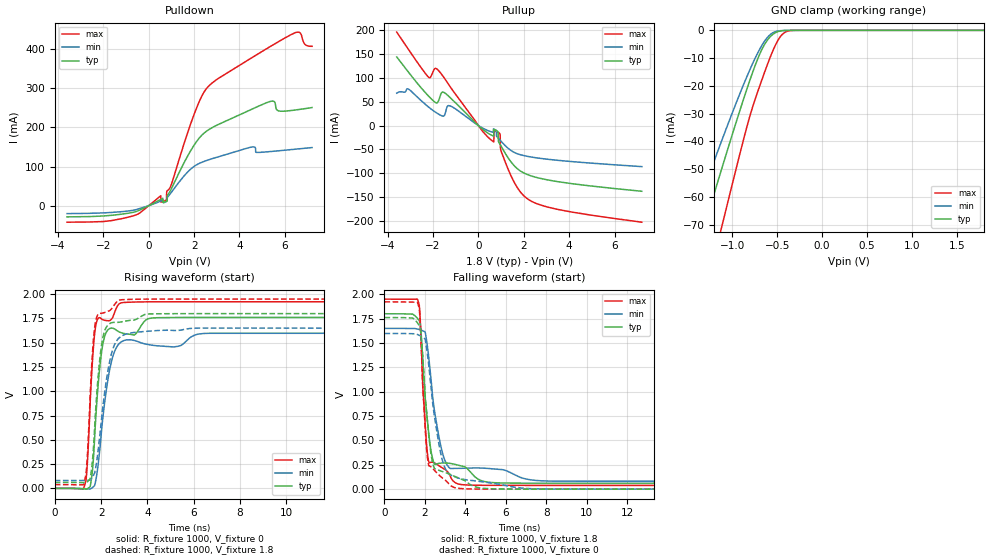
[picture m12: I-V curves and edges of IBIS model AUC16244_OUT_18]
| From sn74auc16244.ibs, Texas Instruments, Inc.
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[Model]   AUC16244_OUT_18
Model_type  3-state
Enable   Active-Low
Vref =   0
Rref =   1000
Cref =   30p
Vmeas =   0.9
| variable   typ   min   max
C_comp   5.46pF   4.88pF   5.67pF
| C_pullup   6.28pF   1.00pF   11.78pF
| C_pulldown   6.14pF   1.75pF   14.74pF
| C_tri-state   5.46pF   4.88pF   5.67pF
[Temperature Range]   40   100   -40
| Ambient temperature   25   85   -40
[Voltage range]   1.8   1.65   1.95
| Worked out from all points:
|   slope of the pulldown table from 0 to 0.27 V, typ, clamps not added: 34.2 ohm
|   slope of the pullup table from 0 to 0.27 V, typ, clamps not added: 24.9 ohm
|   GND clamp passes 1 mA (typ) near -0.53 V on its own axis
|   rising waveform, R_fixture 1000, V_fixture 0: 20-80 % time 343ps typ, 511ps min, 262ps max; typ from 0 V to 1.76 V
|   falling waveform, R_fixture 1000, V_fixture 1.8: 20-80 % time 430ps typ, 642ps min, 291ps max; typ from 1.8 V to 0.061 V
|   rising waveform, R_fixture 1000, V_fixture 1.8: 20-80 % time 339ps typ, 522ps min, 256ps max; typ from 0.061 V to 1.8 V
|   falling waveform, R_fixture 1000, V_fixture 0: 20-80 % time 432ps typ, 649ps min, 291ps max; typ from 1.76 V to 0 V
[GND Clamp]
| AUC16244_OUT_18
|   Voltage   I(typ)   I(min)   I(max)
-3.6V     -322.9mA   -271.3mA   -392.8mA
-1.48V    -89.14mA   -71.99mA   -118.6mA
-1.435V   -84.24mA   -67.93mA   -112.7mA
-1.3V     -69.59mA   -55.85mA   -94.97mA
-1.15V    -53.49mA   -42.68mA   -75.27mA
-1.1V     -48.18mA   -38.36mA   -68.71mA
-830mV    -20.57mA   -16.22mA   -34.06mA
-690mV    -8.335mA   -6.605mA   -19.75mA
-565mV    -1.951mA   -1.255mA   -8.764mA
-490mV    -463.9uA   -245.9uA   -3.576mA
-425mV    -91.38uA   -54.15uA   -985.3uA
1.8V      674.7pA    45.17nA    747.9pA
[Pulldown]
| AUC16244_OUT_18
|   Voltage   I(typ)   I(min)   I(max)
-3.6V     -28.49mA   -20.22mA   -42.08mA
-1.155V   -21.32mA   -15.05mA   -32.66mA
530mV     16.28mA    11.83mA    25.26mA
780mV     11.06mA    10.81mA    14.1mA
800mV     11.7mA     11.72mA    36.72mA
1.955V    150.3mA    98.42mA    225.9mA
2.625V    193.2mA    116.8mA    304mA
4.56V     246.5mA    149.9mA    378.1mA
5.38V     266.4mA    138.3mA    406.9mA
5.71V     242.1mA    140mA      418.2mA
6.445V    244.1mA    144.1mA    441.1mA
7.2V      250.4mA    148.3mA    406.7mA
[Pullup]
| AUC16244_OUT_18
|   Voltage   I(typ)   I(min)   I(max)
-3.6V     143.4mA    67.81mA    195.5mA
-2.21V    62.22mA    39.25mA    101.7mA
-1.955V   50.53mA    30.07mA    117.2mA
-1.505V   68.89mA    20.87mA    99.46mA
-1.25V    58.62mA    41.27mA    81.57mA
405mV     -15.38mA   -10.2mA    -23.47mA
835mV     -11.64mA   -24.19mA   -13.09mA
930mV     -37.45mA   -29.05mA   -16.21mA
980mV     -41.44mA   -31.73mA   -49.64mA
1.31V     -67.6mA    -47.58mA   -91.39mA
2.115V    -101.6mA   -63.91mA   -151.5mA
7.2V      -137.4mA   -85.82mA   -202mA
[Ramp]
| AUC16244_OUT_18
| variable   typ   min   max
dV/dt_r   1.06/3.53E-10   0.96/5.21E-10   1.16/2.72E-10
dV/dt_f   1.04/4.39E-10   0.94/6.57E-10   1.15/2.96E-10
R_load = 1000
[Rising Waveform]
| AUC16244_OUT_18
R_fixture =   1000
C_fixture =   0
L_fixture =   0
V_fixture =   0
V_fixture_min = 0
V_fixture_max = 0
|   Time   V(typ)   V(min)   V(max)
0s        9.675nV    33.63nV    1.209nV
1.325ns   -7.242mV   -3.423mV   61.54mV
1.55ns    46.88mV    -3.891mV   988.5mV
1.72ns    513.6mV    28.82mV    1.59V
1.915ns   1.179V     333.7mV    1.759V
2.13ns    1.545V     838.7mV    1.733V
2.47ns    1.651V     1.328V     1.749V
2.865ns   1.604V     1.508V     1.911V
4.41ns    1.758V     1.469V     1.922V
34.99ns   1.761V     1.597V     1.922V
[Falling Waveform]
| AUC16244_OUT_18
R_fixture =   1000
C_fixture =   0
L_fixture =   0
V_fixture =   1.8
V_fixture_min = 1.65
V_fixture_max = 1.95
|   Time   V(typ)   V(min)   V(max)
0s        1.8V       1.65V      1.95V
1.64ns    1.75V      1.643V     1.942V
1.765ns   1.709V     1.635V     1.745V
1.91ns    1.26V      1.624V     1.003V
2.175ns   595mV      1.375V     291.2mV
2.45ns    266.7mV    832.7mV    270.8mV
2.86ns    268.4mV    377mV      218.1mV
3.66ns    245.3mV    213.5mV    52mV
5.715ns   64mV       202.3mV    38.89mV
34.99ns   61.09mV    81.02mV    38.7mV
[Rising Waveform]
| AUC16244_OUT_18
R_fixture =   1000
C_fixture =   0
L_fixture =   0
V_fixture =   1.8
V_fixture_min = 1.65
V_fixture_max = 1.95
|   Time   V(typ)   V(min)   V(max)
0s        61.05mV    81.01mV    38.68mV
1.235ns   59.36mV    81.82mV    36.94mV
1.375ns   60.93mV    82.92mV    221.2mV
1.525ns   100.9mV    84.6mV     938.1mV
1.735ns   689mV      173.9mV    1.678V
1.895ns   1.211V     438.8mV    1.798V
2.06ns    1.532V     809.7mV    1.805V
2.415ns   1.702V     1.356V     1.84V
2.79ns    1.712V     1.553V     1.94V
34.99ns   1.8V       1.65V      1.95V
[Falling Waveform]
| AUC16244_OUT_18
R_fixture =   1000
C_fixture =   0
L_fixture =   0
V_fixture =   0
V_fixture_min = 0
V_fixture_max = 0
|   Time   V(typ)   V(min)   V(max)
0s        1.761V     1.597V     1.922V
1.64ns    1.703V     1.586V     1.91V
1.795ns   1.6V       1.57V      1.574V
1.915ns   1.289V     1.555V     961.2mV
2.17ns    593.3mV    1.302V     257.6mV
2.425ns   235.9mV    812.2mV    203.6mV
2.81ns    184.6mV    338.3mV    123.4mV
3.475ns   131.3mV    126.1mV    15.34mV
5.585ns   2.262mV    52.78mV    282.6uV
34.99ns   36.42uV    4.075uV    15.87uV
